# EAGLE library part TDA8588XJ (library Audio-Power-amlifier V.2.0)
I2C-bus controlled 4 ´ 50 Watt power amplifier and multiple voltage regulator
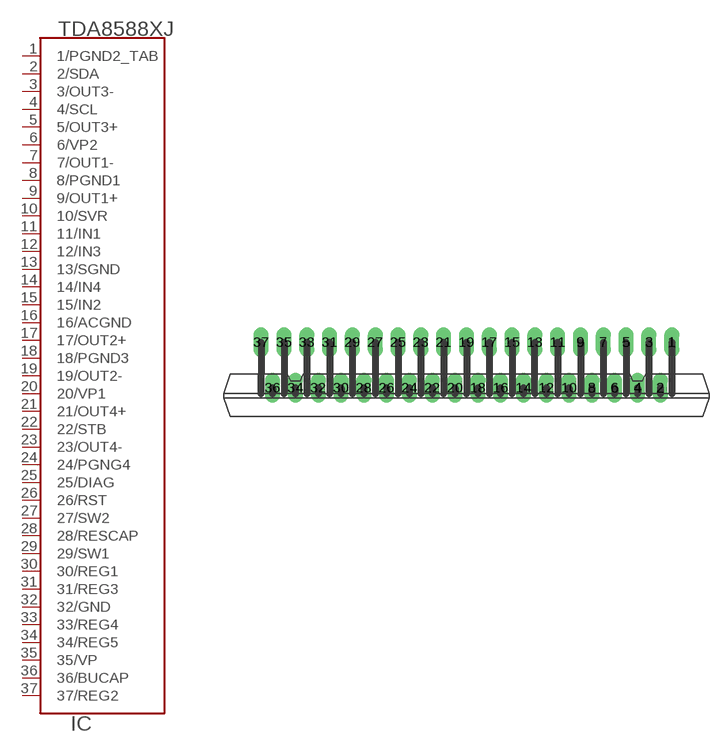
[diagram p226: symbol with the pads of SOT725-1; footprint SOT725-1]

Designator prefix IC

## TDA8588XJ  [SOT725-1]
1  1/PGND2_TAB  pwr
2  2/SDA  out
3  3/OUT3-  out
4  4/SCL  in
5  5/OUT3+  out
6  6/VP2  pwr
7  7/OUT1-  out
8  8/PGND1  pwr
9  9/OUT1+  out
10  10/SVR
11  11/IN1  in
12  12/IN3  in
13  13/SGND  pwr
14  14/IN4  in
15  15/IN2  in
16  16/ACGND  pwr
17  17/OUT2+  out
18  18/PGND3  pwr
19  19/OUT2-  out
20  20/VP1  pwr
21  21/OUT4+  out
22  22/STB  in
23  23/OUT4-  out
24  24/PGNG4  pwr
25  25/DIAG  out
26  26/RST  out
27  27/SW2  out
28  28/RESCAP
29  29/SW1  in
30  30/REG1  out
31  31/REG3  out
32  32/GND  pwr
33  33/REG4  out
34  34/REG5  out
35  35/VP  pwr
36  36/BUCAP  in
37  37/REG2  out

## Footprint SOT725-1 (pad centres in mm)
drill 0.8 long: 1 18,4; 2 17,0; 3 16,4; 4 15,0; 5 14,4; 6 13,0; 7 12,4; 8 11,0; 9 10,4; 10 9,0; 11 8,4; 12 7,0; 13 6,4; 14 5,0; 15 4,4; 16 3,0; 17 2,4; 18 1,0; 19 0,4; 20 -1,0; 21 -2,4; 22 -3,0; 23 -4,4; 24 -5,0; 25 -6,4; 26 -7,0; 27 -8,4; 28 -9,0; 29 -10,4; 30 -11,0; 31 -12,4; 32 -13,0; 33 -14,4; 34 -15,0; 35 -16,4; 36 -17,0; 37 -18,4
